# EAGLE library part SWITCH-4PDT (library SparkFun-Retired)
For use with a push-button switch made by CnK components.
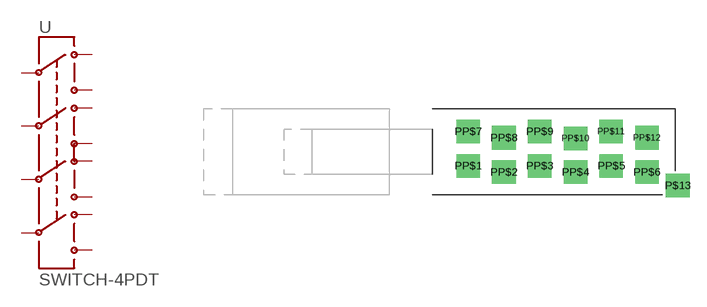
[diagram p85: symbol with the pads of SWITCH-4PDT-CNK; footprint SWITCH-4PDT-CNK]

Designator prefix -

## SWITCH-4PDTCNK_LOCK (PROD_ID: SWCH-09564)  [SWITCH-4PDT-CNK]
PP$1  1
PP$2  2
PP$3  3
PP$4  4
PP$5  5
PP$6  6
PP$7  7
PP$8  8
PP$9  9
PP$10  10
PP$11  11
PP$12  12

## Footprint SWITCH-4PDT-CNK (pad centres in mm)
drill 1.4 square: P$13 0.203,-2.997; PP$1 -18.415,-1.245; PP$2 -15.24,-1.803; PP$3 -12.065,-1.245; PP$4 -8.89,-1.803; PP$5 -5.715,-1.245; PP$6 -2.54,-1.803; PP$7 -18.415,1.803; PP$8 -15.24,1.245; PP$9 -12.065,1.803; PP$10 -8.89,1.194; PP$11 -5.715,1.803; PP$12 -2.54,1.245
